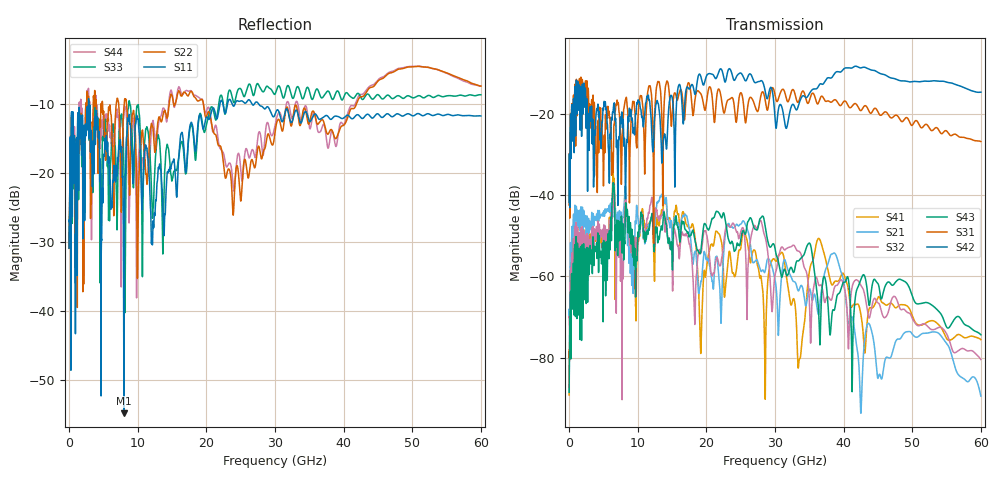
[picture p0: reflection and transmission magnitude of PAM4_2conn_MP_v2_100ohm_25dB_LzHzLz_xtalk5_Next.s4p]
! Info: Touchstone file created by Circ.  Input file=FAB50GbE_2conn_Midplane_Examax_Topo2_v2_100ohm_25dB_LzHzLz.circ
# Hz S RI R 50
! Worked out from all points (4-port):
!   6000 points, 10 MHz to 60 GHz, reference 50 ohm
!   strongest paths, dB at 10 MHz, 15.01 GHz, 30.01 GHz, 45.01 GHz, 60 GHz:
!     S42: -41.8, -15.8, -21.2, -9.7, -14.6
!     S31: -42.4, -20.5, -15.2, -19.5, -26.8
!     S43: -88.6, -55.0, -53.1, -61.8, -74.4
!     S32: -70.1, -55.5, -59.6, -66.5, -80.5
!     S21: -69.8, -50.6, -60.8, -85.1, -89.5
!     S41: -89.2, -49.1, -56.0, -65.2, -75.6
!   lowest |S11| = -54.9 dB at 8 GHz (marker M1), VSWR 1.00, Z = 50.1 + j0.1 ohm
!   |S11| at or under -10 dB: start of sweep to 2.81 GHz; 2.876 GHz to 21.97 GHz (19.1 GHz wide, 154 % of centre); 27.62 GHz to end of sweep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
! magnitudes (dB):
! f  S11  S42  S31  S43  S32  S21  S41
! 10 MHz  -30.9  -41.8  -42.4  -88.6  -70.1  -69.8  -89.2
! 1.28 GHz  -11.3  -12.0  -11.9  -54.8  -49.6  -44.1  -50.3
! 8 GHz  -54.9  -27.8  -18.6  -53.2  -49.1  -43.0  -49.2
! 31 GHz  -12.6  -18.3  -14.0  -60.2  -52.7  -59.2  -54.1
! 33.55 GHz  -12.3  -17.2  -16.5  -56.0  -53.9  -63.1  -80.4
! 36.37 GHz  -12.2  -13.0  -17.1  -69.0  -62.1  -69.2  -50.6
! 60 GHz  -11.7  -14.6  -26.8  -74.4  -80.5  -89.5  -75.6
